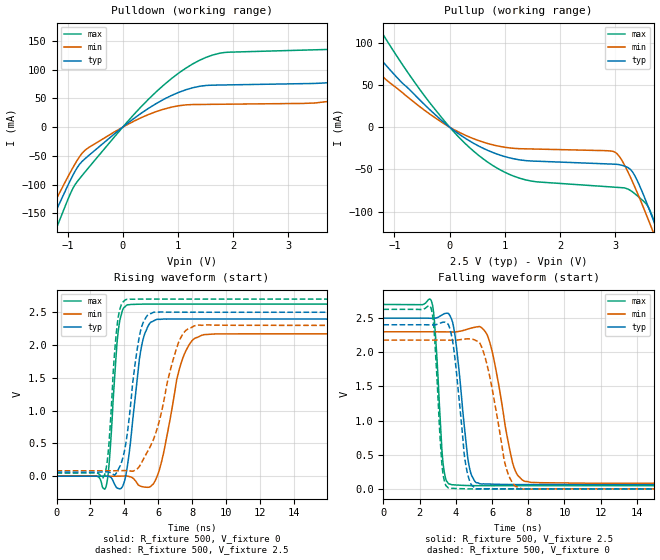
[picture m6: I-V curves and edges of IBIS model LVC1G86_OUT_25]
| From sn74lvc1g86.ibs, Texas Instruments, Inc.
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[Model]   LVC1G86_OUT_25
Model_type  Output
Vref =   0
Rref =   500
Cref =   30p
Vmeas =   1.25
| variable   typ   min   max
C_comp   9.70pF   6.17pF   14.55pF
| C_pullup   9.39pF   6.17pF   11.05pF
| C_pulldown   10.00pF   6.54pF   14.55pF
[Temperature Range]   40   100   -40
| Ambient temperature   25   85   -40
[Voltage range]   2.5   2.3   2.7
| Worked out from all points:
|   slope of the pulldown table from 0 to 0.375 V, typ, clamps not added: 13.9 ohm
|   slope of the pullup table from 0 to 0.375 V, typ, clamps not added: 22.2 ohm
|   rising waveform, R_fixture 500, V_fixture 0: 20-80 % time 626ps typ, 987ps min, 397ps max; typ from 0 V to 2.4 V
|   falling waveform, R_fixture 500, V_fixture 2.5: 20-80 % time 555ps typ, 884ps min, 334ps max; typ from 2.5 V to 0.063 V
|   rising waveform, R_fixture 500, V_fixture 2.5: 20-80 % time 689ps typ, 1.31ns min, 407ps max; typ from 0.063 V to 2.5 V
|   falling waveform, R_fixture 500, V_fixture 0: 20-80 % time 530ps typ, 870ps min, 332ps max; typ from 2.4 V to 0 V
[Pulldown]
| LVC1G86_OUT_25
|   Voltage   I(typ)   I(min)   I(max)
-5V       -943.1mA   -850.1mA   -1.095A
-1.535V   -215.9mA   -188.9mA   -259.6mA
-1.165V   -136.9mA   -118.2mA   -167.3mA
-705mV    -56.93mA   -42.25mA   -80.73mA
50mV      3.852mA    2.688mA    5.583mA
1.745V    73.38mA    39.87mA    128.6mA
3.855V    79.22mA    47.11mA    135.9mA
5.285V    133.6mA    89.67mA    197.1mA
5.595V    150.4mA    47.44mA    219.9mA
5.945V    165.8mA    44.61mA    248.2mA
6.55V     82.98mA    45.06mA    293.4mA
10V       87.5mA     48.06mA    154.1mA
[Pullup]
| LVC1G86_OUT_25
|   Voltage   I(typ)   I(min)   I(max)
-5V       425.2mA    340.3mA    588.3mA
-2.245V   161.9mA    127mA      227.3mA
-1.805V   124.5mA    97.03mA    175.5mA
-1.345V   87.72mA    67.74mA    124.4mA
-95mV     5.052mA    3.755mA    7.344mA
690mV     -27.49mA   -19.35mA   -41.39mA
1.475V    -40.11mA   -25.83mA   -63.76mA
2.99V     -43.86mA   -29.39mA   -71.05mA
3.305V    -52.13mA   -63.23mA   -76.14mA
3.665V    -105.3mA   -120mA     -103.8mA
3.785V    -126.3mA   -140.1mA   -125.1mA
10V       -1.372A    -1.3A      -1.508A
[Ramp]
| LVC1G86_OUT_25
| variable   typ   min   max
dV/dt_r   1.55/7.12E-10   1.40/1.15E-09   1.69/4.31E-10
dV/dt_f   1.50/5.92E-10   1.38/9.68E-10   1.64/3.50E-10
R_load = 500
[Rising Waveform]
| LVC1G86_OUT_25
R_fixture =   500
C_fixture =   0
L_fixture =   0
V_fixture =   0
V_fixture_min = 0
V_fixture_max = 0
|   Time   V(typ)   V(min)   V(max)
0s        129pV      6.161nV    605.2pV
2.9ns     3.027mV    -38.45uV   -173.7mV
3.115ns   -4.566mV   5.817uV    230.4mV
3.64ns    -185.9mV   840.1uV    2.209V
4.2ns     187.9mV    601.4uV    2.615V
5.03ns    1.999V     -156.6mV   2.624V
5.925ns   2.391V     -8.716mV   2.625V
7.395ns   2.398V     1.76V      2.624V
8.695ns   2.397V     2.159V     2.624V
50ns      2.396V     2.17V      2.624V
[Falling Waveform]
| LVC1G86_OUT_25
R_fixture =   500
C_fixture =   0
L_fixture =   0
V_fixture =   2.5
V_fixture_min = 2.3
V_fixture_max = 2.7
|   Time   V(typ)   V(min)   V(max)
0s        2.5V       2.3V       2.7V
2.65ns    2.497V     2.3V       2.75V
3.3ns     2.556V     2.299V     363.8mV
3.77ns    2.481V     2.297V     61.57mV
4.705ns   376.1mV    2.343V     49.26mV
5.355ns   74.19mV    2.372V     47.04mV
6.005ns   69.88mV    2.013V     46.9mV
7.14ns    63.98mV    376.2mV    47.25mV
7.835ns   63.05mV    109.2mV    47.42mV
50ns      63.46mV    83.31mV    47.5mV
[Rising Waveform]
| LVC1G86_OUT_25
R_fixture =   500
C_fixture =   0
L_fixture =   0
V_fixture =   2.5
V_fixture_min = 2.3
V_fixture_max = 2.7
|   Time   V(typ)   V(min)   V(max)
0s        63.44mV    83.27mV    47.49mV
2.84ns    65.54mV    83.23mV    24mV
3.075ns   63.63mV    83.29mV    443.5mV
3.585ns   73.08mV    83.79mV    2.324V
4.12ns    552.1mV    86.25mV    2.696V
4.72ns    1.867V     105.2mV    2.7V
5.155ns   2.367V     274mV      2.701V
7.195ns   2.501V     2.037V     2.7V
8.265ns   2.501V     2.302V     2.7V
50ns      2.5V       2.3V       2.7V
[Falling Waveform]
| LVC1G86_OUT_25
R_fixture =   500
C_fixture =   0
L_fixture =   0
V_fixture =   0
V_fixture_min = 0
V_fixture_max = 0
|   Time   V(typ)   V(min)   V(max)
0s        2.403V     2.179V     2.628V
2.63ns    2.401V     2.179V     2.648V
2.82ns    2.401V     2.179V     2.244V
3.24ns    2.437V     2.178V     337.9mV
3.605ns   2.395V     2.177V     14.39mV
4.555ns   343.7mV    2.195V     1.592mV
5.16ns    1.022mV    2.165V     -278.2uV
6.815ns   365uV      277.9mV    -188.8uV
7.69ns    -309.2uV   -1.209mV   -33.16uV
50ns      20.65uV    35.05uV    11.84uV
